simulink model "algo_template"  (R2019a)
settings: configuration reference "configurationSettings" (kept in a data dictionary, not in this file)
undefined symbols (not defined in the file or in its folder): algo_template_fp, algo_template_tp, ProductionState, QualityTag, signal1, signal2, Value

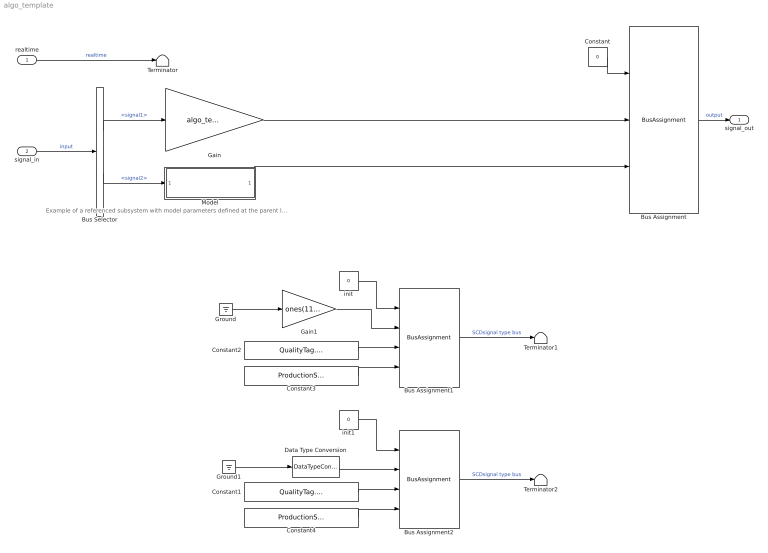
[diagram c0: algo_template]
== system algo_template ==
  note: Example of a referenced subsystem with model parameters defined at the parent level
  realtime : Inport  OutDataTypeStr=single  PortDimensions=1  SampleTime=algo_template_fp.timing.dt  Interpolate=off
  signal_in : Inport  Port=2  OutDataTypeStr=Bus: algo_template_inBus  PortDimensions=1  Interpolate=off
  Bus Assignment : BusAssignment  AssignedSignals=signal1,signal2
  Bus Assignment1 : BusAssignment  AssignedSignals=Value,QualityTag,ProductionState
  Bus Assignment2 : BusAssignment  AssignedSignals=Value,QualityTag,ProductionState
  Bus Selector : BusSelector  OutputSignals=signal1,signal2
  Constant : Constant  Value=0  OutDataTypeStr=Bus: algo_template_outBus
  Constant1 : Constant  Value=QualityTag.INVALID  OutDataTypeStr=Enum: QualityTag
  Constant2 : Constant  Value=QualityTag.GOOD  OutDataTypeStr=Enum: QualityTag
  Constant3 : Constant  Value=ProductionState.RUNNING  OutDataTypeStr=Enum: ProductionState
  Constant4 : Constant  Value=ProductionState.OUTDATED  OutDataTypeStr=Enum: ProductionState
  Data Type Conversion : DataTypeConversion  OutDataTypeStr=int32
  Gain : Gain  Gain=algo_template_tp.gain
  Gain1 : Gain  Gain=ones(11,1)
  Ground : Ground
  Ground1 : Ground
  Model : ModelReference  ModelNameDialog=referenced_model_example.slx  ParameterArgumentNames=TP  ParameterArgumentValues=algo_template_tp.refmodel  UsingDefaultArgumentValue=0  SimulationMode=Normal  ModelReferenceVersion=1.15
  Terminator : Terminator
  Terminator1 : Terminator
  Terminator2 : Terminator
  init : Constant  Value=0  OutDataTypeStr=Bus: SCDBus_single_11_Vector
  init1 : Constant  Value=0  OutDataTypeStr=Bus: SCDBus_int32_Scalar
  signal_out : Outport  OutDataTypeStr=Bus: algo_template_outBus
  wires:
  signal_in/1 -> Bus Selector/1  "input"
  Bus Selector/1 -> Gain/1  "<signal1>"
  Constant/1 -> Bus Assignment/1
  realtime/1 -> Terminator/1  "realtime"
  Bus Assignment/1 -> signal_out/1  "output"
  init/1 -> Bus Assignment1/1
  Bus Assignment1/1 -> Terminator1/1  "SCDsignal type bus"
  Constant2/1 -> Bus Assignment1/3
  Constant3/1 -> Bus Assignment1/4
  Gain1/1 -> Bus Assignment1/2
  init1/1 -> Bus Assignment2/1
  Data Type Conversion/1 -> Bus Assignment2/2
  Constant1/1 -> Bus Assignment2/3
  Constant4/1 -> Bus Assignment2/4
  Bus Assignment2/1 -> Terminator2/1  "SCDsignal type bus"
  Model/1 -> Bus Assignment/3
  Ground1/1 -> Data Type Conversion/1
  Ground/1 -> Gain1/1
  Gain/1 -> Bus Assignment/2
  Bus Selector/2 -> Model/1  "<signal2>"
